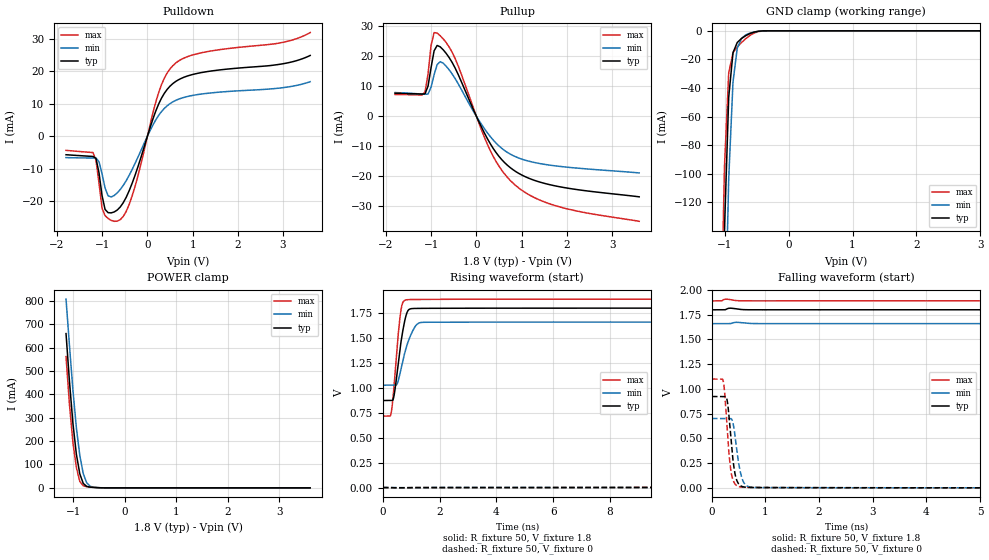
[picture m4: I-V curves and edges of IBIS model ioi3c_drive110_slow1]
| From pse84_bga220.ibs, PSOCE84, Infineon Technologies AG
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[Model] ioi3c_drive110_slow1
Model_type I/O
Enable   Active-High
Vinl  =  0.54
Vinh  =  1.26
Vmeas =  0.9
Cref  =  15e-12
| Capacitance   typ   min   max
C_comp   9.12545e-13 8.87504e-13 9.42456e-13
| Variables   typ   min   max
[GND Clamp Reference]   0   0   0
[POWER Clamp Reference]   1.8   1.66   1.89
[Pulldown Reference]   0   0   0
[Pullup Reference]   1.8   1.66   1.89
[Temperature Range]   25   125   -40
[Voltage Range]   1.8   1.66   1.89
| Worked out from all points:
|   slope of the pulldown table from 0 to 0.27 V, typ, clamps not added: 25.6 ohm
|   slope of the pullup table from 0 to 0.27 V, typ, clamps not added: 33.1 ohm
|   GND clamp passes 1 mA (typ) near -0.55 V on its own axis
|   POWER clamp passes 1 mA (typ) near -0.54 V on its own axis
|   falling waveform, R_fixture 50, V_fixture 1.8: 20-80 % time 94.2ns typ, 141ns min, 54.7ns max; typ from 1.8 V to 0.873 V
|   falling waveform, R_fixture 50, V_fixture 0: 20-80 % time 101ps typ, 117ps min, 92.8ps max; typ from 0.923 V to 0 V
|   rising waveform, R_fixture 50, V_fixture 1.8: 20-80 % time 267ps typ, 376ps min, 209ps max; typ from 0.873 V to 1.8 V
|   rising waveform, R_fixture 50, V_fixture 0: 20-80 % time 99.5ns typ, 151ns min, 59.2ns max; typ from 0 V to 0.923 V
[GND Clamp]
| Voltage   I(typ)   I(min)   I(max)
-1.204V   -737.9mA   -831.5mA   -678.7mA
-1.07V    -303.2mA   -410.8mA   -239.8mA
-1.003V   -139.9mA   -232.2mA   -95.74mA
-936.6mV  -46.51mA   -103.5mA   -29.5mA
-869.7mV  -15.31mA   -35.88mA   -15.36mA
-802.8mV  -8.166mA   -12.13mA   -11.29mA
-735.9mV  -5.335mA   -5.292mA   -8.195mA
-669mV    -3.356mA   -2.85mA    -5.457mA
-535.2mV  -837.9uA   -772uA     -1.483mA
-401.4mV  -47.36uA   -84.85uA   -76.77uA
3.6V      0A         0A         0A
[POWER Clamp]
| Voltage   I(typ)   I(min)   I(max)
-1.137V   660mA      807.5mA    561.8mA
-1.07V    454.5mA    608.2mA    356.2mA
-1.003V   275.7mA    418.4mA    193.6mA
-936.6mV  143.5mA    257.2mA    86.91mA
-869.7mV  59.43mA    137.9mA    27.31mA
-802.8mV  18.8mA     60.93mA    8.704mA
-735.9mV  6.231mA    21.35mA    5.155mA
-669mV    3.127mA    6.887mA    3.44mA
-535.2mV  940.9uA    1.232mA    1.058mA
-334.5mV  16.1uA     59.03uA    7.686uA
3.6V      0A         0A         0A
[Pulldown]
| Voltage   I(typ)   I(min)   I(max)
-1.8V     -5.733mA   -6.615mA   -4.375mA
-1.204V   -6.259mA   -6.731mA   -5.057mA
-1.137V   -6.867mA   -6.731mA   -7.426mA
-1.003V   -18.36mA   -11.66mA   -22.24mA
-936.6mV  -22.64mA   -16.01mA   -24.54mA
-869.7mV  -23.63mA   -18.41mA   -25.44mA
-669mV    -22.83mA   -17.54mA   -26.26mA
-401.4mV  -16.78mA   -12.04mA   -21.01mA
248.3mV   9.926mA    6.426mA    13.46mA
558.6mV   16.21mA    10.57mA    21.74mA
1.117V    19.44mA    12.87mA    25.53mA
3.6V      24.94mA    16.83mA    32.02mA
[Pullup]
| Voltage   I(typ)   I(min)   I(max)
-1.8V     7.685mA    7.95mA     7.309mA
-1.137V   7.524mA    7.374mA    8.102mA
-1.07V    10.09mA    7.426mA    14.14mA
-1.003V   16.26mA    9.76mA     23.64mA
-936.6mV  21.85mA    13.88mA    27.95mA
-869.7mV  23.64mA    17.24mA    27.77mA
-735.9mV  22.21mA    17.75mA    25.87mA
-468.3mV  16.03mA    12.54mA    19.19mA
310.3mV   -9.225mA   -6.807mA   -11.53mA
806.9mV   -17.76mA   -13.05mA   -22.23mA
1.738V    -23.16mA   -16.49mA   -29.74mA
3.6V      -26.83mA   -18.86mA   -34.99mA
[Ramp]
dV/dt_r   0.554027/99.4954n  0.420381/0.150583u  0.660021/59.2218n
dV/dt_f   0.556207/94.244n  0.379694/0.140697u  0.704092/54.7279n
R_load = 50
[Falling Waveform]
R_fixture = 50
V_fixture = 1.8
V_fixture_min = 1.66
V_fixture_max = 1.89
| Time   V(typ)   V(min)   V(max)
0s        1.8V       1.66V      1.89V
9.638ns   1.8V       1.66V      1.868V
19.15ns   1.77V      1.659V     1.683V
37.77ns   1.601V     1.614V     1.339V
62.84ns   1.387V     1.511V     1.042V
93.42ns   1.199V     1.391V     859.8mV
126.9ns   1.069V     1.288V     775.6mV
203.4ns   934.4mV    1.147V     725mV
315.9ns   884.5mV    1.065V     717mV
800ns     873mV      1.027V     716.5mV
[Falling Waveform]
R_fixture = 50
V_fixture = 0
V_fixture_min = 0
V_fixture_max = 0
| Time   V(typ)   V(min)   V(max)
0s        923.4mV    701.3mV    1.1V
212.4ps   923.3mV    701.3mV    1.079V
240.6ps   923.7mV    701.3mV    949.8mV
282.4ps   891.7mV    701.2mV    614.7mV
339.2ps   595.5mV    701.7mV    237.6mV
430.5ps   145.7mV    531.2mV    39.17mV
532.8ps   22.47mV    156.3mV    8.312mV
637.9ps   6.121mV    25.59mV    5.29mV
1.68ns    1.58mV     1.312mV    1.527mV
800ns     9.184nV    627.5nV    3.416nV
[Rising Waveform]
R_fixture = 50
V_fixture = 1.8
V_fixture_min = 1.66
V_fixture_max = 1.89
| Time   V(typ)   V(min)   V(max)
0s        873mV      1.027V     716.5mV
297.3ps   873.1mV    1.027V     753.8mV
401ps     933.1mV    1.027V     1.04V
497.1ps   1.139V     1.036V     1.391V
584.4ps   1.346V     1.119V     1.658V
711.5ps   1.586V     1.28V      1.861V
872.1ps   1.769V     1.449V     1.884V
1.19ns    1.797V     1.634V     1.887V
2.022ns   1.798V     1.659V     1.888V
800ns     1.8V       1.66V      1.89V
[Rising Waveform]
R_fixture = 50
V_fixture = 0
V_fixture_min = 0
V_fixture_max = 0
| Time   V(typ)   V(min)   V(max)
0s        9.15nV     625.6nV    3.411nV
11.81ns   60.4uV     -134.6uV   20.77mV
22ns      35.06mV    4.257mV    183.6mV
45.2ns    231mV      74.75mV    548.2mV
68.19ns   411.6mV    175.4mV    782.9mV
93.27ns   563.8mV    277.6mV    927.8mV
135.1ns   726.8mV    412.7mV    1.034V
212.4ns   857.7mV    562.6mV    1.087V
328.2ns   909.6mV    654.6mV    1.099V
800ns     923.4mV    700.6mV    1.1V
